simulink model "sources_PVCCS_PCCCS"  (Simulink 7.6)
settings: Solver=ode15s  StartTime=0.0  StopTime=10.0  RelTol=1e-3
StopFcn:
  | load signaux.mat
  | plot(x(1,:),x(2,:))
  | title('Sources SPICE : PVCCS et PCCCS')
  | xlabel('temps')
  | grid
libraries: fl_lib x8, elec_lib x4, nesl_utility x3

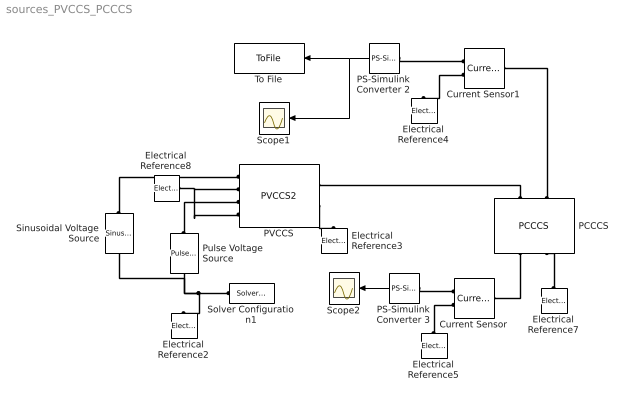
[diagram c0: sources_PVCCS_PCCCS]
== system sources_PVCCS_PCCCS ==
  Current Sensor : fl_lib/Electrical/Electrical Sensors/Current Sensor  DialogController=NetworkEngine.DynNeDlgSource  SystemSampleTime=-1  i1_Log=off  v1_Log=off  LocalVarNames=|i1|v1  LocalVarDescs=|i1|v1  LocalVarLogging=[0 0]
  Current Sensor1 : fl_lib/Electrical/Electrical Sensors/Current Sensor  DialogController=NetworkEngine.DynNeDlgSource  SystemSampleTime=-1  i1_Log=off  v1_Log=off  LocalVarNames=|i1|v1  LocalVarDescs=|i1|v1  LocalVarLogging=[0 0]
  Electrical Reference{2..5,7..8} (6 alike) : fl_lib/Electrical/Electrical Elements/Electrical Reference  DialogController=NetworkEngine.DynNeDlgSource  SystemSampleTime=-1  i_Log=off  LocalVarNames=|i  LocalVarDescs=|i  LocalVarLogging=[]
  PCCCS : elec_lib/Additional Components/SPICE-Compatible Components/Sources/PCCCS  DialogController=NetworkEngine.DynNeDlgSource  SystemSampleTime=-1  PEES=[ 0 0.1 ]  LocalVarLogging=[]
  PS-Simulink Converter 2 : nesl_utility/PS-Simulink Converter  DialogController=NetworkEngine.DynNeUtilDlgSource  SystemSampleTime=-1  PhysicalDomain=network_engine_domain  LeftPortType=input  RightPortType=output  SubClassName=ps_output  Unit=1  AffineConversion=off
  PS-Simulink Converter 3 : nesl_utility/PS-Simulink Converter  DialogController=NetworkEngine.DynNeUtilDlgSource  SystemSampleTime=-1  PhysicalDomain=network_engine_domain  LeftPortType=input  RightPortType=output  SubClassName=ps_output  Unit=1  AffineConversion=off
  PVCCS : elec_lib/Additional Components/SPICE-Compatible Components/Sources/PVCCS2  DialogController=NetworkEngine.DynNeDlgSource  SystemSampleTime=-1  PEES="[  0 1 1 ]"  LocalVarLogging=[]
  Pulse Voltage Source : elec_lib/Additional Components/SPICE-Compatible Components/Sources/Pulse Voltage Source  DialogController=NetworkEngine.DynNeDlgSource  SystemSampleTime=-1  V1=0 V  V2=10 mV  TD=0 s  TR=1e-09 s  TF=1e-09 s  PW=2 s  PER=4 s  voltage_Log=off  LocalVarNames=|voltage  LocalVarDescs=|Voltage (V)  LocalVarLogging=0
  Scope1 : Scope
  Scope2 : Scope
  Sinusoidal Voltage Source : elec_lib/Additional Components/SPICE-Compatible Components/Sources/Sinusoidal Voltage Source  DialogController=NetworkEngine.DynNeDlgSource  SystemSampleTime=-1  VO=0 V  VA=5 mV  FREQ=0.5 Hz  TD=0 s  DF=0 1/s  current_Log=off  voltage_Log=off  power_Log=off  LocalVarNames=|current|voltage|power  LocalVarDescs=|Current (A)|Voltage (V)|Power (W)  LocalVarLogging=[0 0 0]
  Solver Configuration1 : nesl_utility/Solver Configuration  DialogController=NetworkEngine.DynNeUtilDlgSource  SystemSampleTime=-1  PhysicalDomain=network_engine_domain  LeftPortType=input  RightPortType=generic  SubClassName=solver  Accelerate=off  Profile=off  ResidualTolerance=1e-9  MaxNonlinIter=12  MaxModeIter=2  DoFixedCost=off  UseLocalSampling=off  DoDC=off  LinearAlgebra=Sparse  LocalSolverSampleTime=.001  LocalSolverChoice=NE_BACKWARD_EULER_ADVANCER  UseLocalSolver=off
  To File : ToFile  Filename=signaux  MatrixName=x
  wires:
  PS-Simulink Converter 2/1 -> To File/1, Scope1/1
  PS-Simulink Converter 3/1 -> Scope2/1
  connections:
  Solver Configuration1/RConn1 -- Pulse Voltage Source/RConn1 -- Electrical Reference2/LConn1 -- Sinusoidal Voltage Source/RConn1
  Sinusoidal Voltage Source/LConn1 -- PVCCS/LConn1
  PVCCS/RConn2 -- Electrical Reference3/LConn1
  PCCCS/LConn1 -- PVCCS/RConn1
  Electrical Reference7/LConn1 -- PCCCS/RConn2
  PS-Simulink Converter 2/LConn1 -- Current Sensor1/RConn1
  Current Sensor1/RConn2 -- Electrical Reference4/LConn1
  Electrical Reference8/LConn1 -- PVCCS/LConn2 -- PVCCS/LConn4
  Pulse Voltage Source/LConn1 -- PVCCS/LConn3
  PCCCS/LConn2 -- Current Sensor1/LConn1
  PCCCS/RConn1 -- Current Sensor/LConn1
  Electrical Reference5/LConn1 -- Current Sensor/RConn2
  PS-Simulink Converter 3/LConn1 -- Current Sensor/RConn1
